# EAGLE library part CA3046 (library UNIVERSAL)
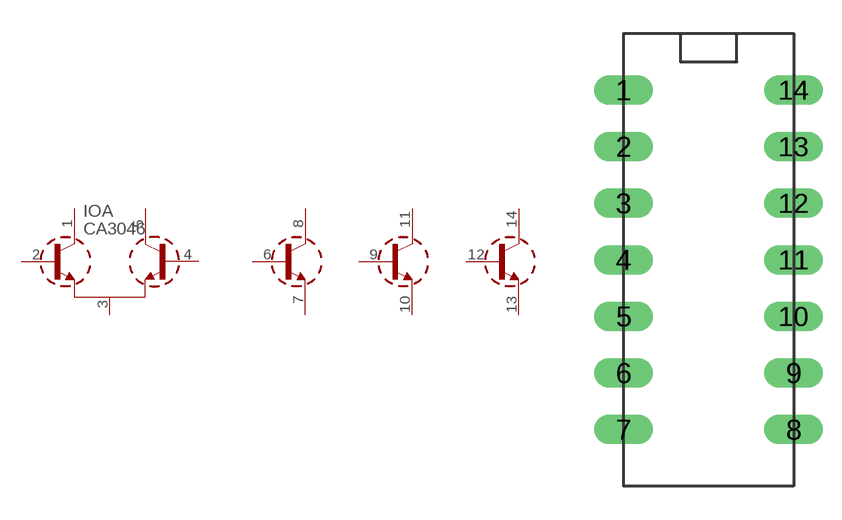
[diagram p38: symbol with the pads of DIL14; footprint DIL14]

Designator prefix IO; gates A=NPNZ B=NPN C=NPN D=NPN

## CA3046  [DIL14]
1  A:AC
2  A:AB
3  A:SE
4  A:BB
5  A:BC
6  B:B
7  B:E
8  B:C
9  C:B
10  C:E
11  C:C
12  D:B
13  D:E
14  D:C

## Footprint DIL14 (pad centres in mm)
drill 0.813 pad 1.092 long: 1 0,0; 2 0,-2.54; 3 0,-5.08; 4 0,-7.62; 5 0,-10.16; 6 0,-12.7; 7 0,-15.24; 8 7.62,-15.24; 9 7.62,-12.7; 10 7.62,-10.16; 11 7.62,-7.62; 12 7.62,-5.08; 13 7.62,-2.54; 14 7.62,0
